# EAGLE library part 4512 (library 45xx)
8-channel DATA SELECTOR Inhibit function corrected - 2005.10.04 librarian@cadsoft.de
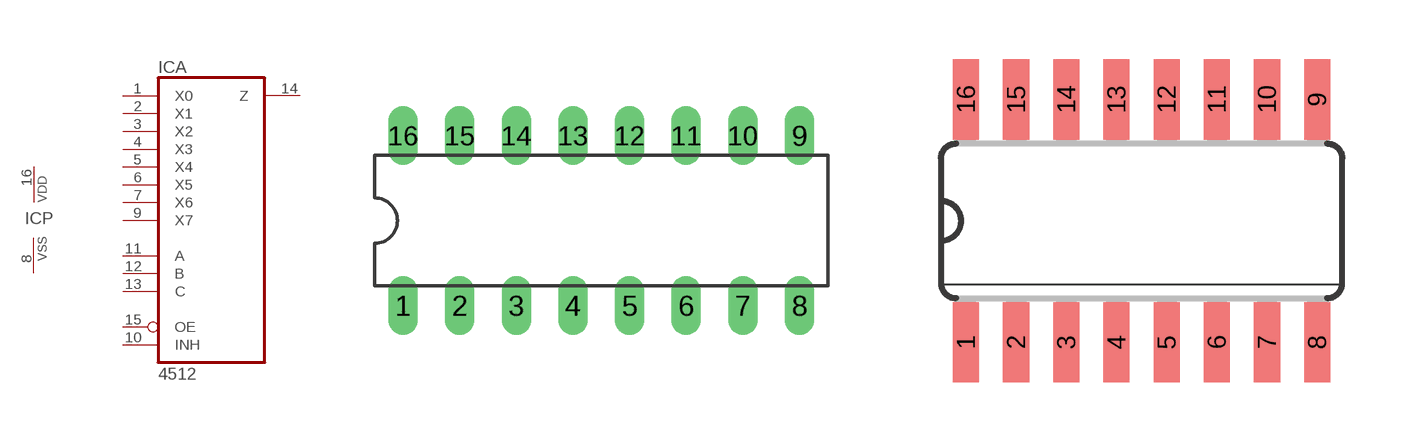
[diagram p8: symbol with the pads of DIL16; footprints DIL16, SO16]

Designator prefix IC; gates A=4512 P=PWRN

## 4512N  [DIL16]
1  A:X0  in
2  A:X1  in
3  A:X2  in
4  A:X3  in
5  A:X4  in
6  A:X5  in
7  A:X6  in
8  P:VSS  pwr
9  A:X7  in
10  A:INH  in
11  A:A  in
12  A:B  in
13  A:C  in
14  A:Z  hiz
15  A:OE  in
16  P:VDD  pwr

## 4512D  [SO16]
Pads as for DIL16

## Footprint DIL16 (pad centres in mm)
Dual In Line Package
drill 0.813 long: 1 -8.89,-3.81; 2 -6.35,-3.81; 3 -3.81,-3.81; 4 -1.27,-3.81; 5 1.27,-3.81; 6 3.81,-3.81; 7 6.35,-3.81; 8 8.89,-3.81; 9 8.89,3.81; 10 6.35,3.81; 11 3.81,3.81; 12 1.27,3.81; 13 -1.27,3.81; 14 -3.81,3.81; 15 -6.35,3.81; 16 -8.89,3.81

## Footprint SO16 (pad centres in mm)
Small Outline package 150 mil
smd 0.66 x 2.032: 1 -4.445,-3.073; 2 -3.175,-3.073; 3 -1.905,-3.073; 4 -0.635,-3.073; 5 0.635,-3.073; 6 1.905,-3.073; 7 3.175,-3.073; 8 4.445,-3.073; 9 4.445,3.073; 10 3.175,3.073; 11 1.905,3.073; 12 0.635,3.073; 13 -0.635,3.073; 14 -1.905,3.073; 15 -3.175,3.073; 16 -4.445,3.073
